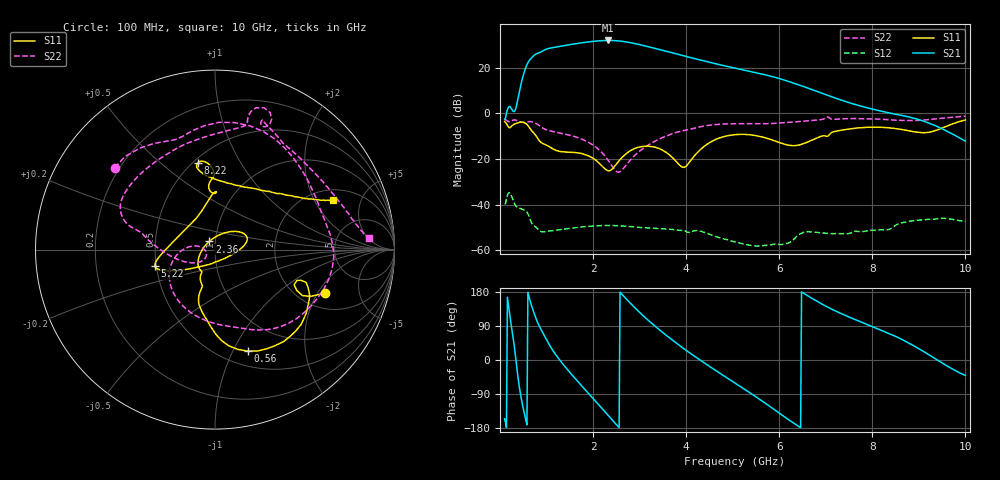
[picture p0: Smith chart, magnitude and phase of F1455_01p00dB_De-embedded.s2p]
! Integrated Device Technology
! Corporate Headquarters
! 6024 Silver Creek Valley Road
! San Jose, CA 95138  USA
! Phone:  1-408-284-8200
! Toll Free:  1-800-223-1366
! Webpage:  http://www.idt.com/
! Timing and RF Division
! 515 Groton Road, Suite 102
! Westford, MA 01886-6024
! Device:  F1455
! Description: 6-bit 0.5 dB Transmit Variable Gain Amplifier
! Frequency:  1400.0 -  2300.00 MHz
! Package:  6x6 mm Thin QFN Plastic Package: 28 pin
! State:  2
! Atten State:  1.0 dB
! Voltage:  +5.00 Volts
! Current:  214.208 mA
! Data:  The device was measured on a the F1455 evaluation board which has
!  individual transmission lines to the RF pins.  Data was collected
!  using a calibrated network analyzer.  The evaluation board was
!  de-embedded using a TRL calibration technique.
!  The reference plane is the edge of the package pin.
!  Pin  1 = CSb
!  Pin  2 = DATA
!  Pin  3 = CLK
!  Pin  4 = RSET
!  Pin  5 = GND
!  Pin  6 = RFIN  = Port 1
!  Pin  7 = GND
!  Pin  8 = NC
!  Pin  9 = NC
!  Pin 10 = NC
!  Pin 11 = NC
!  Pin 12 = NC
!  Pin 13 = NC
!  Pin 14 = /STBY
!  Pin 15 = GND
!  Pin 16 = RFOUT  = Port 2
!  Pin 17 = GND
!  Pin 18 = NC
!  Pin 19 = NC
!  Pin 20 = NC
!  Pin 21 = GND
!  Pin 22 = NC
!  Pin 23 = GND
!  Pin 24 = NC
!  Pin 25 = NC
!  Pin 26 = NC
!  Pin 27 = GND
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# GHz S dB R 50
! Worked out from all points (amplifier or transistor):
!   496 points, 100 MHz to 10 GHz, reference 50 ohm
!   highest |S21| = 31.9 dB at 2.32 GHz (marker M1)
!   |S21| within 3 dB of that: 1.176 GHz to 3.236 GHz (2.061 GHz wide, 93.4 % of centre)
!   unconditionally stable (mu >= 1): start of sweep to end of sweep
!   at 1.74 GHz: K = 4.06, MAG = 31.3 dB, |S12| = -49.8 dB
!   at 5.06 GHz: K = 19.53, MAG = 22.1 dB, |S12| = -56.3 dB
!   at 10 GHz: K = 58.58, MAG = -3.0 dB, |S12| = -47.4 dB
!   S11 on the Smith chart (normalised r, x): 100 MHz: 2.70, -2.31; 560 MHz: 0.66, -1.14; 2.36 GHz: 0.93, +0.09; 5.22 GHz: 0.49, -0.10; 8.22 GHz: 0.53, +0.67; 10 GHz: 2.53, +2.87
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0.1  -3.64 -21.6  -2.55 -154.9  -39.82 39.5  -2.83 140.8
0.4  -4.06 -37.7  7.83 -57.2  -41.36 -110.6  -3.42 50.4
0.56  -4.52 -72.1  20.30 -160.2  -42.83 -164.2  -3.99 15.9
0.7  -8.06 -96.4  24.72 135.7  -48.67 154.9  -3.82 -20.4
0.82  -11.29 -109.3  26.40 95.7  -50.82 137.1  -4.98 -49.7
0.96  -13.57 -110.2  27.78 62.5  -51.86 125.5  -6.89 -73.8
1.14  -15.60 -119.2  28.78 24.4  -51.33 102.9  -7.98 -97.1
1.34  -16.83 -121.0  29.52 -8.8  -50.77 81.7  -8.85 -119.8
1.76  -17.61 -135.1  30.89 -68.8  -49.72 47.4  -11.30 -157.1
2.04  -20.26 -156.3  31.60 -106.8  -49.30 28.6  -14.50 -178.0
2.32  -25.15 140.3  31.91 -145.4  -49.10 11.1  -20.43 168.5
2.36  -25.08 125.0  31.91 -150.9  -49.12 8.8  -21.56 169.4
2.6  -19.81 63.0  31.59 176.3  -49.30 -5.0  -25.25 -150.5
2.9  -15.39 35.0  30.54 137.7  -49.82 -19.3  -18.33 -143.4
3.4  -15.27 10.7  28.07 82.3  -50.47 -38.6  -11.50 -174.5
4.02  -22.75 -94.3  24.80 23.7  -52.07 -64.3  -7.24 166.5
5.06  -9.31 -162.3  19.73 -61.4  -56.34 -96.1  -4.54 148.3
5.22  -9.20 -165.0  19.03 -74.2  -57.23 -96.3  -4.53 143.2
6.7  -11.70 100.9  10.43 162.9  -51.94 -126.9  -3.13 78.1
8.22  -6.15 101.3  0.81 76.8  -51.00 176.5  -2.60 65.4
8.36  -6.36 102.2  0.16 69.7  -50.81 178.5  -2.79 62.2
10  -2.92 22.8  -12.12 -40.6  -47.40 90.9  -1.28 4.5
